DATA_BLOCK "DIVE_DB"
TITLE =
VERSION : 0.1


  STRUCT
   RUN : BOOL ;	//Produzione in corso
   MANUALE : BOOL ;	//Manuale
   ALLARME : BOOL ;	//Allarme
   MANCATO_CARICO : BOOL ;	//Mancato Carico
   MANCATO_SCARICO : BOOL ;	//Mancato Scarico
   PRESENZA_PEZZO : BOOL ;	//Presenza pezzo
   ESITO_OK : BOOL ;	//Pezzo OK
   ESITO_KO : BOOL ;	//Pezzo KO
   SPARE : BOOL ;
   FINE_LAVORO : BOOL ;	//Lavorazione finita
   INIZIO_PALLET : BOOL ;	//Inizio pallet
   FINE_PALLET : BOOL ;	//Fine pallet
   PEZZI_BUONI : BOOL ;	//Segnale pezzo buono
   PEZZI_SCARTO : BOOL ;	//Segnale pezzo scarto
   SPARE_1 : BOOL ;	//Disponibile
   SPARE_2 : BOOL ;	//Disponibile
   CODICE_PALLET : DWORD ;	//Numero codice pallet
   SPARE_DWORD_1 : DWORD ;	//Disponibile
   SPARE_DWORD_2 : DWORD ;	//Disponibile
   SCARTO : BOOL ;	//Pezzo Scarto
   SPARE1 : BOOL ;	//Disponibile
   SPARE2 : BOOL ;	//Disponibile
   SPARE3 : BOOL ;	//Disponibile
   SPARE4 : BOOL ;	//Disponibile
   SPARE5 : BOOL ;	//Disponibile
   SPARE6 : BOOL ;	//Disponibile
   SPARE7 : BOOL ;	//Disponibile
   SPARE8 : BOOL ;	//Disponibile
   SPARE9 : BOOL ;	//Disponibile
   SPARE10 : BOOL ;	//Disponibile
   SPARE11 : BOOL ;	//Disponibile
   SPARE12 : BOOL ;	//Disponibile
   SPARE13 : BOOL ;	//Disponibile
   SPARE14 : BOOL ;	//Disponibile
   SPARE15 : BOOL ;	//Disponibile
   SPARE_DWORD_3 : DWORD ;	//Disponibile
   SPARE_DWORD_4 : DWORD ;	//Disponibile
  END_STRUCT ;
BEGIN
   RUN := FALSE;
   MANUALE := FALSE;
   ALLARME := FALSE;
   MANCATO_CARICO := FALSE;
   MANCATO_SCARICO := FALSE;
   PRESENZA_PEZZO := FALSE;
   ESITO_OK := FALSE;
   ESITO_KO := FALSE;
   SPARE := FALSE;
   FINE_LAVORO := FALSE;
   INIZIO_PALLET := FALSE;
   FINE_PALLET := FALSE;
   PEZZI_BUONI := FALSE;
   PEZZI_SCARTO := FALSE;
   SPARE_1 := FALSE;
   SPARE_2 := FALSE;
   CODICE_PALLET := DW#16#0;
   SPARE_DWORD_1 := DW#16#0;
   SPARE_DWORD_2 := DW#16#0;
   SCARTO := FALSE;
   SPARE1 := FALSE;
   SPARE2 := FALSE;
   SPARE3 := FALSE;
   SPARE4 := FALSE;
   SPARE5 := FALSE;
   SPARE6 := FALSE;
   SPARE7 := FALSE;
   SPARE8 := FALSE;
   SPARE9 := FALSE;
   SPARE10 := FALSE;
   SPARE11 := FALSE;
   SPARE12 := FALSE;
   SPARE13 := FALSE;
   SPARE14 := FALSE;
   SPARE15 := FALSE;
   SPARE_DWORD_3 := DW#16#0;
   SPARE_DWORD_4 := DW#16#0;
END_DATA_BLOCK

FUNCTION "DIVE" : VOID
TITLE =
VERSION : 0.1


VAR_TEMP
  zero : BOOL ;
END_VAR
BEGIN
NETWORK
TITLE =Produzione in corso
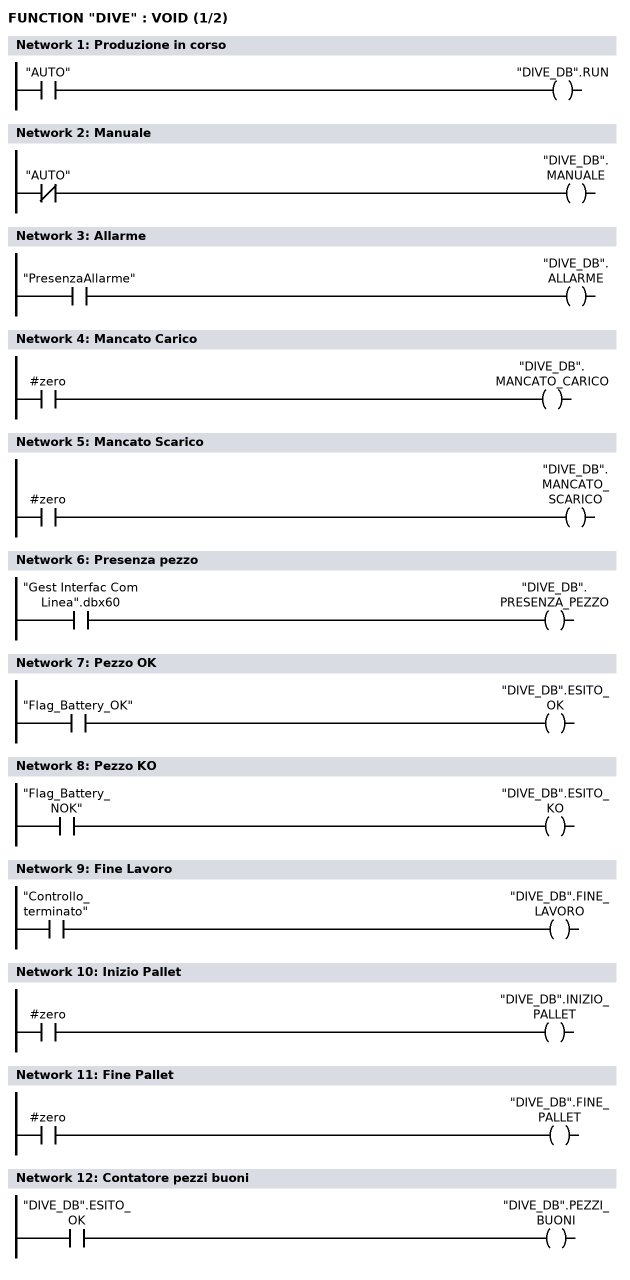
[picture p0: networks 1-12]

      U     "AUTO";
      =     "DIVE_DB".RUN;
NETWORK
TITLE =Manuale

      UN    "AUTO";
      =     "DIVE_DB".MANUALE;
NETWORK
TITLE =Allarme

      U     "PresenzaAllarme";
      =     "DIVE_DB".ALLARME;
NETWORK
TITLE =Mancato Carico

      U     #zero;
      =     "DIVE_DB".MANCATO_CARICO;
NETWORK
TITLE =Mancato Scarico

      U     #zero;
      =     "DIVE_DB".MANCATO_SCARICO;
NETWORK
TITLE =Presenza pezzo

      U     "Gest Interfac Com Linea".dbx60;
      =     "DIVE_DB".PRESENZA_PEZZO;
NETWORK
TITLE =Pezzo OK

      U     "Flag_Battery_OK";
      =     "DIVE_DB".ESITO_OK;
NETWORK
TITLE =Pezzo KO

      U     "Flag_Battery_NOK";
      =     "DIVE_DB".ESITO_KO;
NETWORK
TITLE =Fine Lavoro

      U     "Controllo_terminato";
      =     "DIVE_DB".FINE_LAVORO;
NETWORK
TITLE =Inizio Pallet

      U     #zero;
      =     "DIVE_DB".INIZIO_PALLET;
NETWORK
TITLE =Fine Pallet

      U     #zero;
      =     "DIVE_DB".FINE_PALLET;
NETWORK
TITLE =Contatore pezzi buoni

      U     "DIVE_DB".ESITO_OK;
      =     "DIVE_DB".PEZZI_BUONI;
NETWORK
TITLE =Contatore pezzi scarto
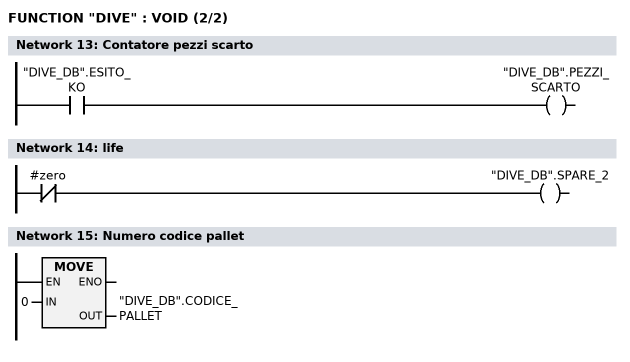
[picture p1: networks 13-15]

      U     "DIVE_DB".ESITO_KO;
      =     "DIVE_DB".PEZZI_SCARTO;
NETWORK
TITLE =life

      UN    #zero;
      =     "DIVE_DB".SPARE_2;
NETWORK
TITLE =Numero codice pallet

      L     0;
      T     "DIVE_DB".CODICE_PALLET;
      NOP   0;
END_FUNCTION

